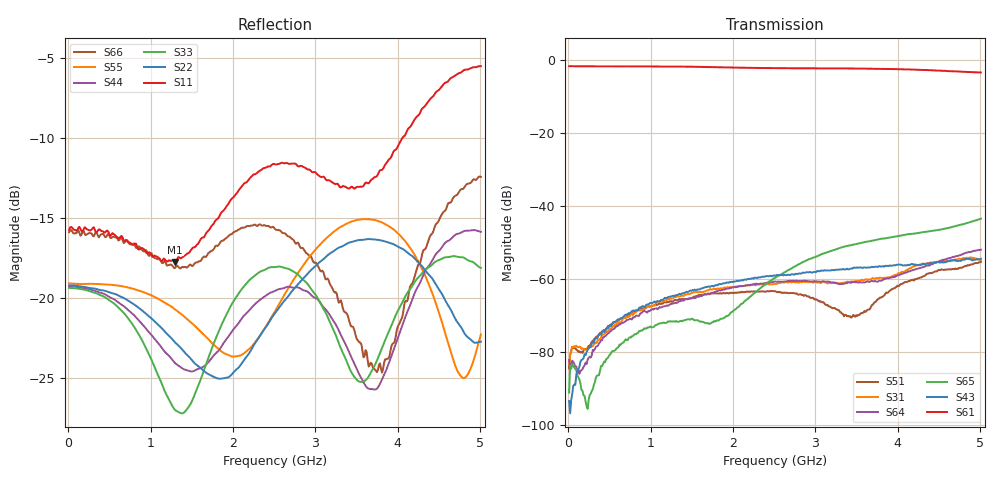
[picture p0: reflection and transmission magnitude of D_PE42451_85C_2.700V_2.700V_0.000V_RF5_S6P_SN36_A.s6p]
! Device ID: PE42451
! Serial: 36
! Insertion: A
! Temp: 85C
! VDD: 2.700
! Control_Hi: 100.000
! Control_Lo: 0.000
! Logic State: RF5
! Port 1: RFC
! Port 2: RF1
! Port 3: RF2
! Port 4: RF3
! Port 5: RF4
! Port 6: RF5
! V1 = 2.70
! V2 = 0.00
! V3 = 2.70
! V4 = 0.00
! IDD: 1.155040e-05
#  Hz  S  RI  R  50
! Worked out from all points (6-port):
!   401 points, 10 MHz to 5.01 GHz, reference 50 ohm
!   strongest paths, dB at 10 MHz, 1.26 GHz, 2.51 GHz, 3.76 GHz, 5.01 GHz:
!     S61: -1.7, -1.8, -2.3, -2.4, -3.5
!     S43: -93.5, -64.7, -59.2, -56.8, -54.5
!     S65: -91.3, -71.7, -59.7, -49.2, -43.6
!     S64: -82.3, -66.9, -60.7, -60.8, -52.0
!     S31: -83.5, -65.4, -61.4, -59.9, -54.9
!     S51: -84.6, -66.4, -63.4, -65.6, -55.4
!   lowest |S11| = -17.8 dB at 1.298 GHz (marker M1), VSWR 1.30, Z = 55.4 - j12.6 ohm
!   |S11| at or under -10 dB: start of sweep to 4.059 GHz
